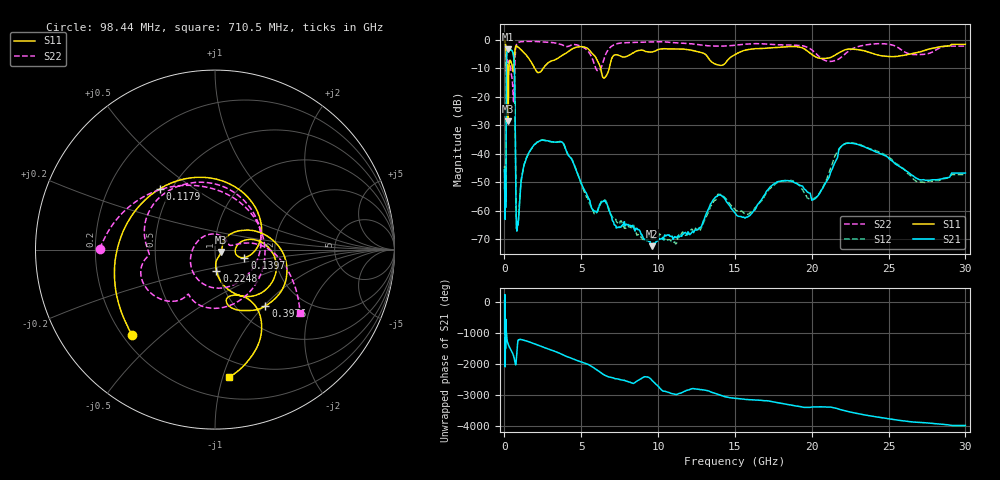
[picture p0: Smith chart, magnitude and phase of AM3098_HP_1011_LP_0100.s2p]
! Date/Time: Thu, Feb 28, 2019 8:43 AM
! Network Analyzer: Agilent Technologies E8364B Rev: A.07.50.67
! Sweep from 0.010 to 30.000 GHz, 1601 Points, Sweep Type: LOG
! Power Supply: 5.023 V, 0.002 A
# Hz S DB R 50
!freq MagS11 AngS11 MagS21 AngS21 MagS12 AngS12 MagS22 AngS22
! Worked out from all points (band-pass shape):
!   1601 points, 10 MHz to 30 GHz, reference 50 ohm
!   highest |S21| = -3.41 dB at 241.1 MHz (marker M1); lowest = -72.5 dB at 9.586 GHz (marker M2)
!   |S21| within 3 dB of the highest: 136.5 MHz to 606.7 MHz (470.2 MHz wide, 127 % of centre)
!   lowest |S11| = -28.7 dB at 239.9 MHz (marker M3), VSWR 1.08, Z = 53.5 - j1.38 ohm
!   |S11| at or under -10 dB: 200.7 MHz to 292.1 MHz (91.4 MHz wide, 37.1 % of centre); 1.959 GHz to 2.53 GHz (570.4 MHz wide, 25.4 % of centre); 6.252 GHz to 6.824 GHz (572.7 MHz wide, 8.76 % of centre)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
!   |S22| runs from -21.8 to -0.5 dB; largest |S21 - S12| = 0.011
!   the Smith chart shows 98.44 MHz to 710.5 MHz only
!   S11 on the Smith chart (normalised r, x): 98.44 MHz: 0.24, -0.40; 117.9 MHz: 0.43, +0.37; 139.7 MHz: 1.38, -0.13; 224.8 MHz: 0.99, -0.24; 397.6 MHz: 1.34, -1.02; 710.5 MHz: 0.36, -1.05
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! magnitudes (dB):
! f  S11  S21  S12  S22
! 10 MHz  -0.3  -46.6  -45.0  -0.5
! 38.04 MHz  -0.4  -61.5  -59.0  -0.7
! 98.44 MHz  -3.6  -50.3  -52.4  -3.9
! 117.9 MHz  -6.8  -20.6  -20.6  -10.7
! 139.7 MHz  -15.4  -5.8  -5.7  -10.6
! 144.7 MHz  -18.3  -5.1  -5.1  -10.8
! 186.8 MHz  -8.7  -4.0  -4.0  -7.1
! 224.8 MHz  -18.3  -3.5  -3.5  -8.5
! 239.9 MHz  -28.7  -3.4  -3.4  -8.7
! 241.1 MHz  -28.7  -3.4  -3.4  -8.7
! 397.6 MHz  -7.5  -3.6  -3.6  -9.7
! 550.5 MHz  -11.0  -4.6  -4.6  -18.6
! 649.3 MHz  -6.4  -10.9  -10.9  -14.7
! 710.5 MHz  -2.9  -36.3  -35.9  -4.6
! 809.2 MHz  -2.3  -66.7  -65.1  -1.5
! 2.084 GHz  -11.1  -36.3  -36.2  -0.7
! 3.76 GHz  -5.5  -36.0  -36.0  -1.9
! 7.926 GHz  -6.0  -64.8  -66.2  -1.1
! 9.586 GHz  -4.4  -72.5  -70.5  -0.9
! 20.1 GHz  -5.6  -56.2  -55.8  -4.1
! 22.56 GHz  -3.4  -36.4  -36.3  -3.5
! 30 GHz  -1.7  -46.9  -47.4  -2.3
